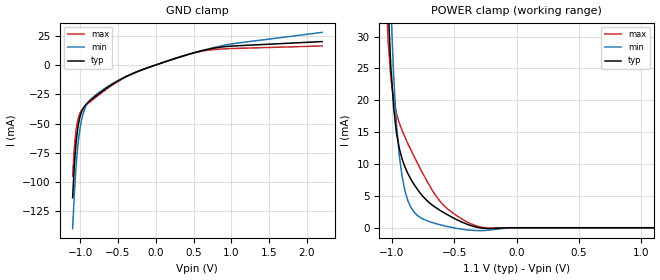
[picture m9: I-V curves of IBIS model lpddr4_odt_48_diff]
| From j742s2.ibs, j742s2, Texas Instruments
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|   Model lpddr4_odt_48_diff
[Model] lpddr4_odt_48_diff
Model_type Input
Polarity   Non-Inverting
Enable   Active-High
Vinl =  0.113V
Vinh =  0.253V
C_comp   1.679pF   1.501pF   1.938pF
[Model Spec]
Vinh   0.253V   0.247V   0.265V
Vinl   0.113V   0.107V   0.125V
[Temperature Range]   25.000   0.125k   -40.000
[Voltage Range]   1.100V   1.060V   1.170V
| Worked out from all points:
|   GND clamp passes 1 mA (typ) near -0.04 V on its own axis
|   POWER clamp passes 1 mA (typ) near -0.45 V on its own axis
[GND_clamp]
|Voltage   I(typ)   I(min)   I(max)
-1.1V     -113.3mA   -139.7mA   -95mA
-1.077V   -85.25mA   -109.4mA   -70.15mA
-1.054V   -65.89mA   -86.08mA   -55.09mA
-1.031V   -53.33mA   -68.84mA   -46.62mA
-1.008V   -45.46mA   -56.48mA   -41.87mA
-985mV    -40.51mA   -47.81mA   -39mA
-940mV    -35mA      -37.46mA   -35.47mA
-802mV    -26.9mA    -25.96mA   -28.05mA
-321mV    -7.781mA   -7.629mA   -7.969mA
527mV     10.78mA    10.68mA    10.61mA
963mV     15.87mA    17.49mA    13.9mA
2.2V      19.95mA    27.78mA    16.19mA
[POWER_clamp]
|Voltage   I(typ)   I(min)   I(max)
-1.1V     113.7mA    140.6mA    93.47mA
-1.031V   35.58mA    50.63mA    29.76mA
-1.008V   25.2mA     34.82mA    23.58mA
-985mV    18.85mA    23.82mA    20.08mA
-963mV    14.95mA    16.34mA    17.96mA
-940mV    12.44mA    11.32mA    16.43mA
-917mV    10.76mA    7.976mA    15.25mA
-871mV    8.491mA    4.244mA    13.18mA
-779mV    5.598mA    1.706mA    9.539mA
-596mV    2.524mA    383.2uA    3.754mA
-298mV    9.874uA    -444.5uA   157uA
1.1V      0A         0A         0A
